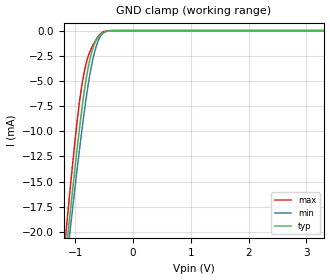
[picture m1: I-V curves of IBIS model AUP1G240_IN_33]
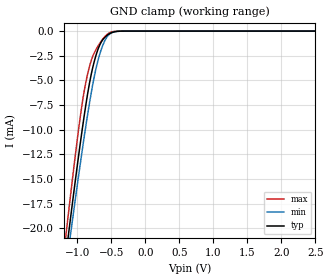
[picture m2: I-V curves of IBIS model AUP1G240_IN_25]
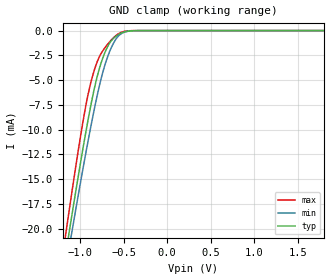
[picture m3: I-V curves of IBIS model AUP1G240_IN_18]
| TEXAS INSTRUMENTS INCORPORATED
| Standard Linear and Logic Group
| IBIS Model of SN74AUP1G240
| LOW-POWER SINGLE BUFFER/DRIVER WITH 3-STATE OUTPUT
| This file contains package information for the following:
|  SOT 5-pin (DCK) package as [Component] AUP1G240_DCK
|  SOT 5-pin (DBV) package as [Component] AUP1G240_DBV
|  DSBGA 5-pin (YEP_YZP) package as [Component] AUP1G240_YEP_YZP
|  XSON 5-pin (DPW) package as [Component] AUP1G240_DPW
| This device can be powered at the following Vccs:
|  3.3 volt Vcc
|  2.5 volt Vcc
|  1.8 volt Vcc
|  1.5 volt Vcc
|  1.2 volt Vcc
|  0.8 volt Vcc
| This file provides unique models under the [Model Selector] for each Vcc.
| For operation at a specific Vcc, select the appropriate model after each
| [Model Selector] keyword.
[IBIS Ver]   3.2
[Comment char]  |_char
[File Name]   sn74aup1g240.ibs
[File Rev]   1.2 | x_die
[Date]   09/19/2017
[Source]   Data created from TI-SPICE simulations.
   Texas Instruments Incorporated.
   Analog-eLab, HPA
   12500 TI Blvd
   Dallas, TX -75243
   For Support e-mail: odt-pfmodeling@list.ti.com
[Notes]   The following is an IBIS list for the AUP1G240.
   - FILE REV HISTORY
   - 1.1 Release IBIS file on 03/30/05
   - 1.2 DPW package update released on 09/19/2017
   - Power clamp data deleted as there is no power-clamp diode.
   - Non-monotonic data in pullup due to special output circuit.
[Disclaimer]  This model is designed as an aid for customers of Texas Instruments
 TI and its licensors and suppliers make no warranties, either expressed
 or implied, with respect to this  model, including the warranties of
 merchantability or fitness for a particular purpose.
 The model is provided solely on an "as is" basis. The entire risk as to
 its quality and performance is with the customer.
[Copyright] (C)Copyright 2017 Texas Instruments Incorporated.
   All rights reserved.
| Component AUP1G240_DCK 5-pin SOT
[Component]   AUP1G240_DCK
[Manufacturer]   Texas Instruments, Inc.
[Package]
|   typ   min   max
R_pkg   2.000e-02   1.700e-02   2.500e-02
L_pkg   9.980e-10   8.810e-10   1.069e-09
C_pkg   1.460e-13   1.180e-13   2.050e-13
[Pin]   signal_name   model_name   R_pin   L_pin   C_pin
1   NOE   AUP1G240_NOE   1.900e-02   1.069e-09   1.620e-13
2   A   AUP1G240_IN   1.800e-02   8.810e-10   1.210e-13
3   GND   GND   1.700e-02   1.031e-09   2.050e-13
4   Y   AUP1G240_OUT   2.000e-02   9.600e-10   1.240e-13
5   VCC   POWER   2.500e-02   1.049e-09   1.180e-13
| Component AUP1G240_DBV 5-pin SOT
[Component]   AUP1G240_DBV
[Manufacturer]   Texas Instruments, Inc.
[Package]
|   typ   min   max
R_pkg   2.500e-02   2.100e-02   2.900e-02
L_pkg   1.529e-09   1.312e-09   1.906e-09
C_pkg   1.560e-13   1.100e-13   2.400e-13
[Pin]   signal_name   model_name   R_pin   L_pin   C_pin
1   NOE   AUP1G240_NOE   2.100e-02   1.511e-09   1.440e-13
2   A   AUP1G240_IN   2.300e-02   1.312e-09   1.380e-13
3   GND   GND   2.900e-02   1.906e-09   2.400e-13
4   Y   AUP1G240_OUT   2.600e-02   1.541e-09   1.500e-13
5   VCC   POWER   2.500e-02   1.374e-09   1.100e-13
| Component AUP1G240_YEP_YZP 5-pin DSBGA
[Component]   AUP1G240_YEP_YZP
[Manufacturer]   Texas Instruments, Inc.
[Package]
|   typ   min   max
R_pkg   1.000e-03   1.000e-03   1.000e-03
L_pkg   2.100e-11   2.100e-11   2.100e-11
C_pkg   4.600e-14   4.500e-14   4.700e-14
[Pin]   signal_name   model_name   R_pin   L_pin   C_pin
1   NOE   AUP1G240_NOE   1.000e-03   2.100e-11   4.600e-14
2   A   AUP1G240_IN   1.000e-03   2.100e-11   4.700e-14
3   GND   GND   1.000e-03   2.100e-11   4.600e-14
4   Y   AUP1G240_OUT   1.000e-03   2.100e-11   4.500e-14
5   VCC   POWER   1.000e-03   2.100e-11   4.500e-14
| Component LVC1G38D_DPW 5-pin X2SON
[Component]   LVC1G38D_DPW
[Manufacturer]   Texas Instruments, Inc.
[Package]
|   typ   min   max
R_pkg   0.0364   0.0010   0.0518
L_pkg   0.2978n   0.0346n   0.4435n
C_pkg   0.0978p   0.0741p   0.1133p
[Pin]   signal_name   model_name   R_pin   L_pin   C_pin
1   D   LVC1G38D_IN   0.04116   0.30011n   0.10160p
2   CLK   LVC1G38D_IN   0.05181   0.44351n   0.11332p
3   GND   GND   0.00103   0.03456n   0.07412p
4   Q   LVC1G38D_OUT   0.04142   0.34311n   0.10148p
5   VCC   POWER   0.04662   0.36767n   0.09844p
| Model AUP1G240_IN
[Model Selector]   AUP1G240_IN
AUP1G240_IN_33   3.3 volt Vcc
AUP1G240_IN_25   2.5 volt Vcc
AUP1G240_IN_18   1.8 volt Vcc
AUP1G240_IN_15   1.5 volt Vcc
AUP1G240_IN_12   1.2 volt Vcc
AUP1G240_IN_08   0.8 volt Vcc
| Model AUP1G240_NOE
[Model Selector]   AUP1G240_NOE
AUP1G240_NOE_33   3.3 volt Vcc
AUP1G240_NOE_25   2.5 volt Vcc
AUP1G240_NOE_18   1.8 volt Vcc
AUP1G240_NOE_15   1.5 volt Vcc
AUP1G240_NOE_12   1.2 volt Vcc
AUP1G240_NOE_08   0.8 volt Vcc
| Model AUP1G240_OUT
[Model Selector]   AUP1G240_OUT
AUP1G240_OUT_33   3.3 volt Vcc
AUP1G240_OUT_25   2.5 volt Vcc
AUP1G240_OUT_18   1.8 volt Vcc
AUP1G240_OUT_15   1.5 volt Vcc
AUP1G240_OUT_12   1.2 volt Vcc
AUP1G240_OUT_08   0.8 volt Vcc
| Models and submodels in the file (18): AUP1G240_IN_33 (Input), AUP1G240_IN_25 (Input), AUP1G240_IN_18 (Input), AUP1G240_IN_15 (Input), AUP1G240_IN_12 (Input), AUP1G240_IN_08 (Input), AUP1G240_NOE_33 (Input), AUP1G240_NOE_25 (Input), AUP1G240_NOE_18 (Input), AUP1G240_NOE_15 (Input), AUP1G240_NOE_12 (Input), AUP1G240_NOE_08 (Input), AUP1G240_OUT_33 (3-state), AUP1G240_OUT_25 (3-state), AUP1G240_OUT_18 (3-state), AUP1G240_OUT_15 (3-state), AUP1G240_OUT_12 (3-state), AUP1G240_OUT_08 (3-state)
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[Model]   AUP1G240_IN_33
Model_type  Input
Vinl=0.9
Vinh=2
| variable   typ   min   max
C_comp   1.40pF   1.15pF   1.78pF
[Temperature Range]   40   100   -40
| Ambient temperature   25   85   -40
[Voltage range]   3.3   3   3.6
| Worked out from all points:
|   GND clamp passes 1 mA (typ) near -0.64 V on its own axis
[GND Clamp]
| AUP1G240_IN_33
|   Voltage   I(typ)   I(min)   I(max)
-3.6V     -171.6mA   -163.5mA   -181.1mA
-1.16V    -22.22mA   -23.69mA   -20.18mA
-1.11V    -19.45mA   -21.09mA   -17.19mA
-1.085V   -18.08mA   -19.81mA   -15.71mA
-940mV    -10.5mA    -12.6mA    -7.822mA
-890mV    -8.117mA   -10.26mA   -5.698mA
-835mV    -5.768mA   -7.825mA   -3.925mA
-755mV    -3.153mA   -4.717mA   -2.255mA
-675mV    -1.463mA   -2.419mA   -1.277mA
-595mV    -617.7uA   -945.8uA   -546.7uA
-515mV    -215.4uA   -248.8uA   -134.4uA
3.3V      132.2pA    540.4pA    36.28pA
[Model]   AUP1G240_IN_25
Model_type  Input
Vinl=0.7
Vinh=1.6
| variable   typ   min   max
C_comp   1.44pF   1.20pF   1.76pF
[Temperature Range]   40   100   -40
| Ambient temperature   25   85   -40
[Voltage range]   2.5   2.3   2.7
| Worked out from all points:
|   GND clamp passes 1 mA (typ) near -0.64 V on its own axis
[GND Clamp]
| AUP1G240_IN_25
|   Voltage   I(typ)   I(min)   I(max)
-3.6V     -171.6mA   -163.5mA   -181.1mA
-1.165V   -22.5mA    -23.95mA   -20.48mA
-1.115V   -19.72mA   -21.35mA   -17.49mA
-1.09V    -18.36mA   -20.06mA   -16.01mA
-945mV    -10.75mA   -12.84mA   -8.061mA
-890mV    -8.117mA   -10.26mA   -5.698mA
-835mV    -5.768mA   -7.825mA   -3.925mA
-760mV    -3.287mA   -4.89mA    -2.329mA
-675mV    -1.463mA   -2.419mA   -1.277mA
-595mV    -617.7uA   -945.8uA   -546.7uA
-520mV    -233.1uA   -272.6uA   -149.9uA
2.5V      104.3pA    491.9pA    26.71pA
[Model]   AUP1G240_IN_18
Model_type  Input
Vinl=0.6825
Vinh=1.0725
| variable   typ   min   max
C_comp   1.49pF   1.27pF   1.76pF
[Temperature Range]   40   100   -40
| Ambient temperature   25   85   -40
[Voltage range]   1.8   1.65   1.95
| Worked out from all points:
|   GND clamp passes 1 mA (typ) near -0.64 V on its own axis
[GND Clamp]
| AUP1G240_IN_18
|   Voltage   I(typ)   I(min)   I(max)
-3.6V     -171.6mA   -163.5mA   -181.1mA
-1.16V    -22.22mA   -23.69mA   -20.18mA
-1.135V   -20.83mA   -22.39mA   -18.68mA
-1.11V    -19.45mA   -21.09mA   -17.19mA
-1.09V    -18.36mA   -20.06mA   -16.01mA
-960mV    -11.5mA    -13.57mA   -8.799mA
-850mV    -6.372mA   -8.471mA   -4.359mA
-780mV    -3.86mA    -5.615mA   -2.659mA
-710mV    -2.096mA   -3.313mA   -1.67mA
-625mV    -855.5uA   -1.409mA   -788.9uA
-540mV    -313.2uA   -390uA     -224.9uA
1.8V      83.14pA    451.3pA    18.98pA
